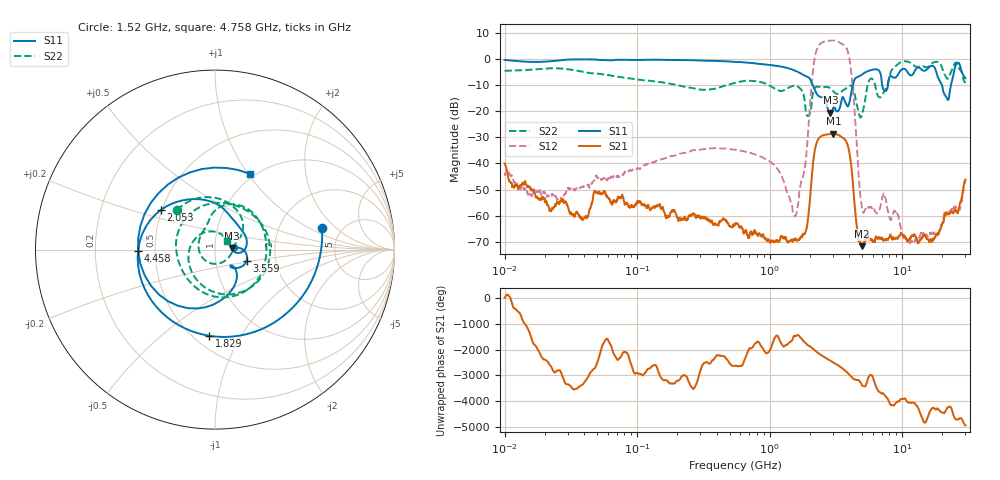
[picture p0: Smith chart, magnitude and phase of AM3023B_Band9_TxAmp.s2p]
# Hz S DB R 50.0
!freq dBS11 angS11 dBS21 angS21 dBS12 angS12 dBS22 angS22
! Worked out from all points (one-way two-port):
!   1601 points, 10 MHz to 30 GHz, reference 50 ohm
!   highest |S21| = -28.67 dB at 3.032 GHz (marker M1); lowest = -71.7 dB at 4.952 GHz (marker M2)
!   lowest |S11| = -20.6 dB at 2.87 GHz (marker M3), VSWR 1.21, Z = 60.2 + j1.04 ohm
!   |S11| at or under -10 dB: 2.108 GHz to 4.251 GHz (2.143 GHz wide, 67.4 % of centre); 7.057 GHz to 7.819 GHz (761.6 MHz wide, 10.2 % of centre); 19.94 GHz to 23.36 GHz (3.426 GHz wide, 15.8 % of centre)
!   |S22| runs from -22.5 to -0.9 dB; largest |S21 - S12| = 2.3
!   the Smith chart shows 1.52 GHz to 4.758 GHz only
!   S11 on the Smith chart (normalised r, x): 1.52 GHz: 3.54, +1.37; 1.829 GHz: 0.59, -0.74; 2.053 GHz: 0.49, +0.25; 3.559 GHz: 1.41, -0.18; 4.458 GHz: 0.40, -0.01; 4.758 GHz: 0.95, +1.02
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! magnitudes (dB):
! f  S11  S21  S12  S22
! 10 MHz  -0.4  -40.0  -44.0  -4.6
! 38.04 MHz  -0.2  -60.9  -49.0  -4.8
! 49.35 MHz  -0.3  -51.1  -44.6  -5.6
! 144.7 MHz  -0.4  -56.0  -38.8  -8.8
! 547.7 MHz  -1.2  -63.3  -34.8  -9.2
! 1.082 GHz  -2.5  -69.9  -40.6  -11.3
! 1.52 GHz  -4.3  -69.3  -59.3  -10.3
! 1.829 GHz  -6.4  -66.8  -42.7  -15.1
! 2.053 GHz  -8.5  -48.9  -12.4  -19.1
! 2.084 GHz  -9.4  -44.6  -8.6  -15.9
! 2.87 GHz  -20.6  -28.7  7.0  -11.3
! 3.032 GHz  -18.4  -28.7  7.0  -12.5
! 3.559 GHz  -14.6  -30.2  5.5  -12.2
! 4.013 GHz  -16.3  -36.4  -0.5  -10.3
! 4.458 GHz  -7.4  -60.2  -25.9  -15.5
! 4.758 GHz  -6.7  -69.9  -48.5  -21.7
! 4.952 GHz  -6.1  -71.7  -56.7  -21.7
! 5.725 GHz  -4.4  -69.1  -56.7  -7.8
! 7.926 GHz  -7.7  -68.5  -59.6  -8.1
! 18.19 GHz  -5.5  -66.9  -66.6  -1.1
! 21.78 GHz  -15.1  -59.2  -58.9  -7.5
! 30 GHz  -7.4  -46.3  -46.2  -9.3
